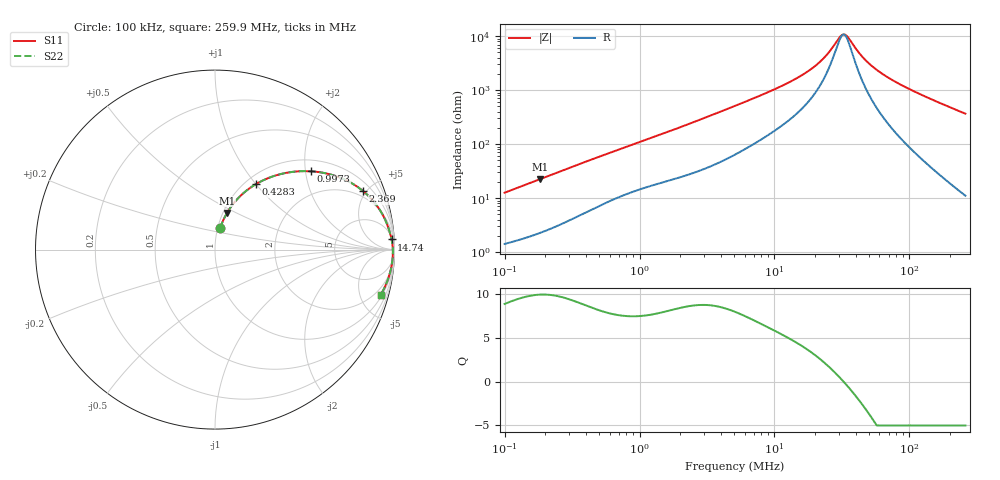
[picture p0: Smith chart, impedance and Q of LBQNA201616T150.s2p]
! LBQNA201616T150  S-PARAMETER MODEL  ( General Type )
! Model Generated by TAIYO YUDEN Corporation (http://www.ty-top.com)
! Version 1.0
! TAIYO YUDEN Control No. 191025NI43SB-FBB
! Copyright(c) 2019 TAIYO YUDEN CO.,LTD. All Rights Reserved.
! Product Description (link to TY-COMPAS)
! https://ds.yuden.co.jp/TYCOMPAS/or/detail?pn=LBQNA201616T150K&u=M
! Products Name : Inductors
! Characteristics :
!  Inductance : 15 uH , SRF(min) : 28 MHz , DC Resistance(max) : 0.91 Ohm
!  Rated Current : Saturation :210 mA , Temp Rise : 220 mA (20 degC)
!  Case Size : 2.0 x 1.6 / 0.079 x 0.063 [mm/inch] , Thickness : 1.6 / 0.063 [mm/inch]
!  (Conditions: Temperature = 25 degC , DC Bias Current/Voltage = 0A / 0V)
! External Node Assignments :
!  1  o---GGG---o  2
! GND o---------o GND
! Frequency Range : 0.1MHz  -  259.929867MHz  [ 402 STEP ]
# MHz S RI R 50
! Freq[MHz].  S11 Real  S11 Imag  S21 Real  S21 Imag  S12 Real  S12 Imag  S22 Real  S22 Imag
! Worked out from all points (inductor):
!   401 points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, 100 kHz to 259.9 MHz, reference 50 ohm
!   read as one part in series: L = 19.7 uH near 104 kHz
!   highest Q = 9.91 at 183.9 kHz (marker M1), where L = 19.4 uH
!   self-resonance near 32.35 MHz
!   S11 on the Smith chart (normalised r, x): 100 kHz: 1.03, +0.25; 428.3 kHz: 1.12, +1.00; 997.3 kHz: 1.29, +2.14; 2.369 MHz: 1.56, +4.78; 14.74 MHz: 8, +33; 259.9 MHz: 1.22, -7.31
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0.1  0.0286 0.1195  0.9714 -0.1195  0.9714 -0.1195  0.0286 0.1195
0.183929  0.0671 0.2048  0.9329 -0.2048  0.9329 -0.2048  0.0671 0.2048
0.37324  0.1899 0.3398  0.8101 -0.3398  0.8101 -0.3398  0.1899 0.3398
0.4283  0.228 0.3648  0.772 -0.3648  0.772 -0.3648  0.228 0.3648
0.660033  0.3742 0.4228  0.6258 -0.4228  0.6258 -0.4228  0.3742 0.4228
0.997345  0.5348 0.4363  0.4652 -0.4363  0.4652 -0.4363  0.5348 0.4363
1.393082  0.6627 0.413  0.3373 -0.413  0.3373 -0.413  0.6627 0.413
2.368534  0.8263 0.3252  0.1737 -0.3252  0.1737 -0.3252  0.8263 0.3252
5.098332  0.9422 0.1787  0.0578 -0.1787  0.0578 -0.1787  0.9422 0.1787
9.563494  0.974 0.0959  0.026 -0.0959  0.026 -0.0959  0.974 0.0959
14.73784  0.9837 0.0563  0.0163 -0.0563  0.0163 -0.0563  0.9837 0.0563
19.02902  0.9872 0.0367  0.0128 -0.0367  0.0128 -0.0367  0.9872 0.0367
24.09141  0.9894 0.0201  0.0106 -0.0201  0.0106 -0.0201  0.9894 0.0201
30.50056  0.9906 0.00421  0.0094 -0.00421  0.0094 -0.00421  0.9906 0.00421
32.99563  0.9908 -0.00107  0.00915 0.00107  0.00915 0.00107  0.9908 -0.00107
34.99999  0.991 -0.00504  0.00903 0.00504  0.00903 0.00504  0.991 -0.00504
42.60291  0.9911 -0.0186  0.00894 0.0186  0.00894 0.0186  0.9911 -0.0186
48.88766  0.9908 -0.0285  0.00919 0.0285  0.00919 0.0285  0.9908 -0.0285
58.34901  0.99 -0.042  0.00996 0.042  0.00996 0.042  0.99 -0.042
71.02397  0.9885 -0.0586  0.0115 0.0586  0.0115 0.0586  0.9885 -0.0586
123.153  0.9778 -0.1186  0.0222 0.1186  0.0222 0.1186  0.9778 -0.1186
259.9299  0.924 -0.2504  0.076 0.2504  0.076 0.2504  0.924 -0.2504
